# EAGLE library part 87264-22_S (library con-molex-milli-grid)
RECEPTACAL
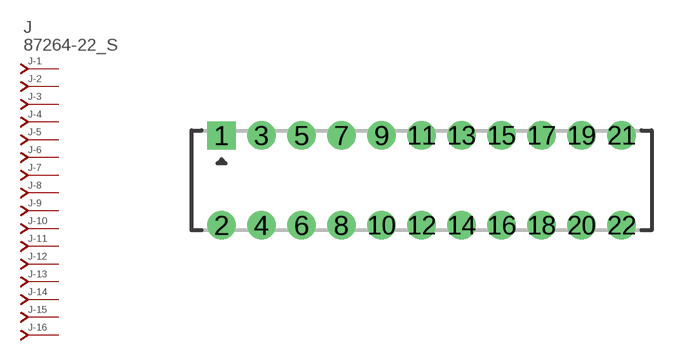
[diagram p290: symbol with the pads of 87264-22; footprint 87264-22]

Designator prefix J; gates -1=J-NV -2=J-N -3=J-N -4=J-N -5=J-N -6=J-N -7=J-N -8=J-N -9=J-N -10=J-N -11=J-N -12=J-N -13=J-N -14=J-N -15=J-N -16=J-N -17=J-N -18=J-N -19=J-N -20=J-N -21=J-N -22=J-N

## 87264-22_S  [87264-22]
1  -1:J  pas
2  -2:J  pas
3  -3:J  pas
4  -4:J  pas
5  -5:J  pas
6  -6:J  pas
7  -7:J  pas
8  -8:J  pas
9  -9:J  pas
10  -10:J  pas
11  -11:J  pas
12  -12:J  pas
13  -13:J  pas
14  -14:J  pas
15  -15:J  pas
16  -16:J  pas
17  -17:J  pas
18  -18:J  pas
19  -19:J  pas
20  -20:J  pas
21  -21:J  pas
22  -22:J  pas

## Footprint 87264-22 (pad centres in mm)
RECEPTACAL Dual Row, Side Entry
drill 0.914 square: 1 -10,2.25
drill 0.914: 2 -10,-2.25; 3 -8,2.25; 4 -8,-2.25; 5 -6,2.25; 6 -6,-2.25; 7 -4,2.25; 8 -4,-2.25; 9 -2,2.25; 10 -2,-2.25; 11 0,2.25; 12 0,-2.25; 13 2,2.25; 14 2,-2.25; 15 4,2.25; 16 4,-2.25; 17 6,2.25; 18 6,-2.25; 19 8,2.25; 20 8,-2.25; 21 10,2.25; 22 10,-2.25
